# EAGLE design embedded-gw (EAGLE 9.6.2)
AUTHOR: Neal Jackson; REV: B; TITLE: Embedded GW

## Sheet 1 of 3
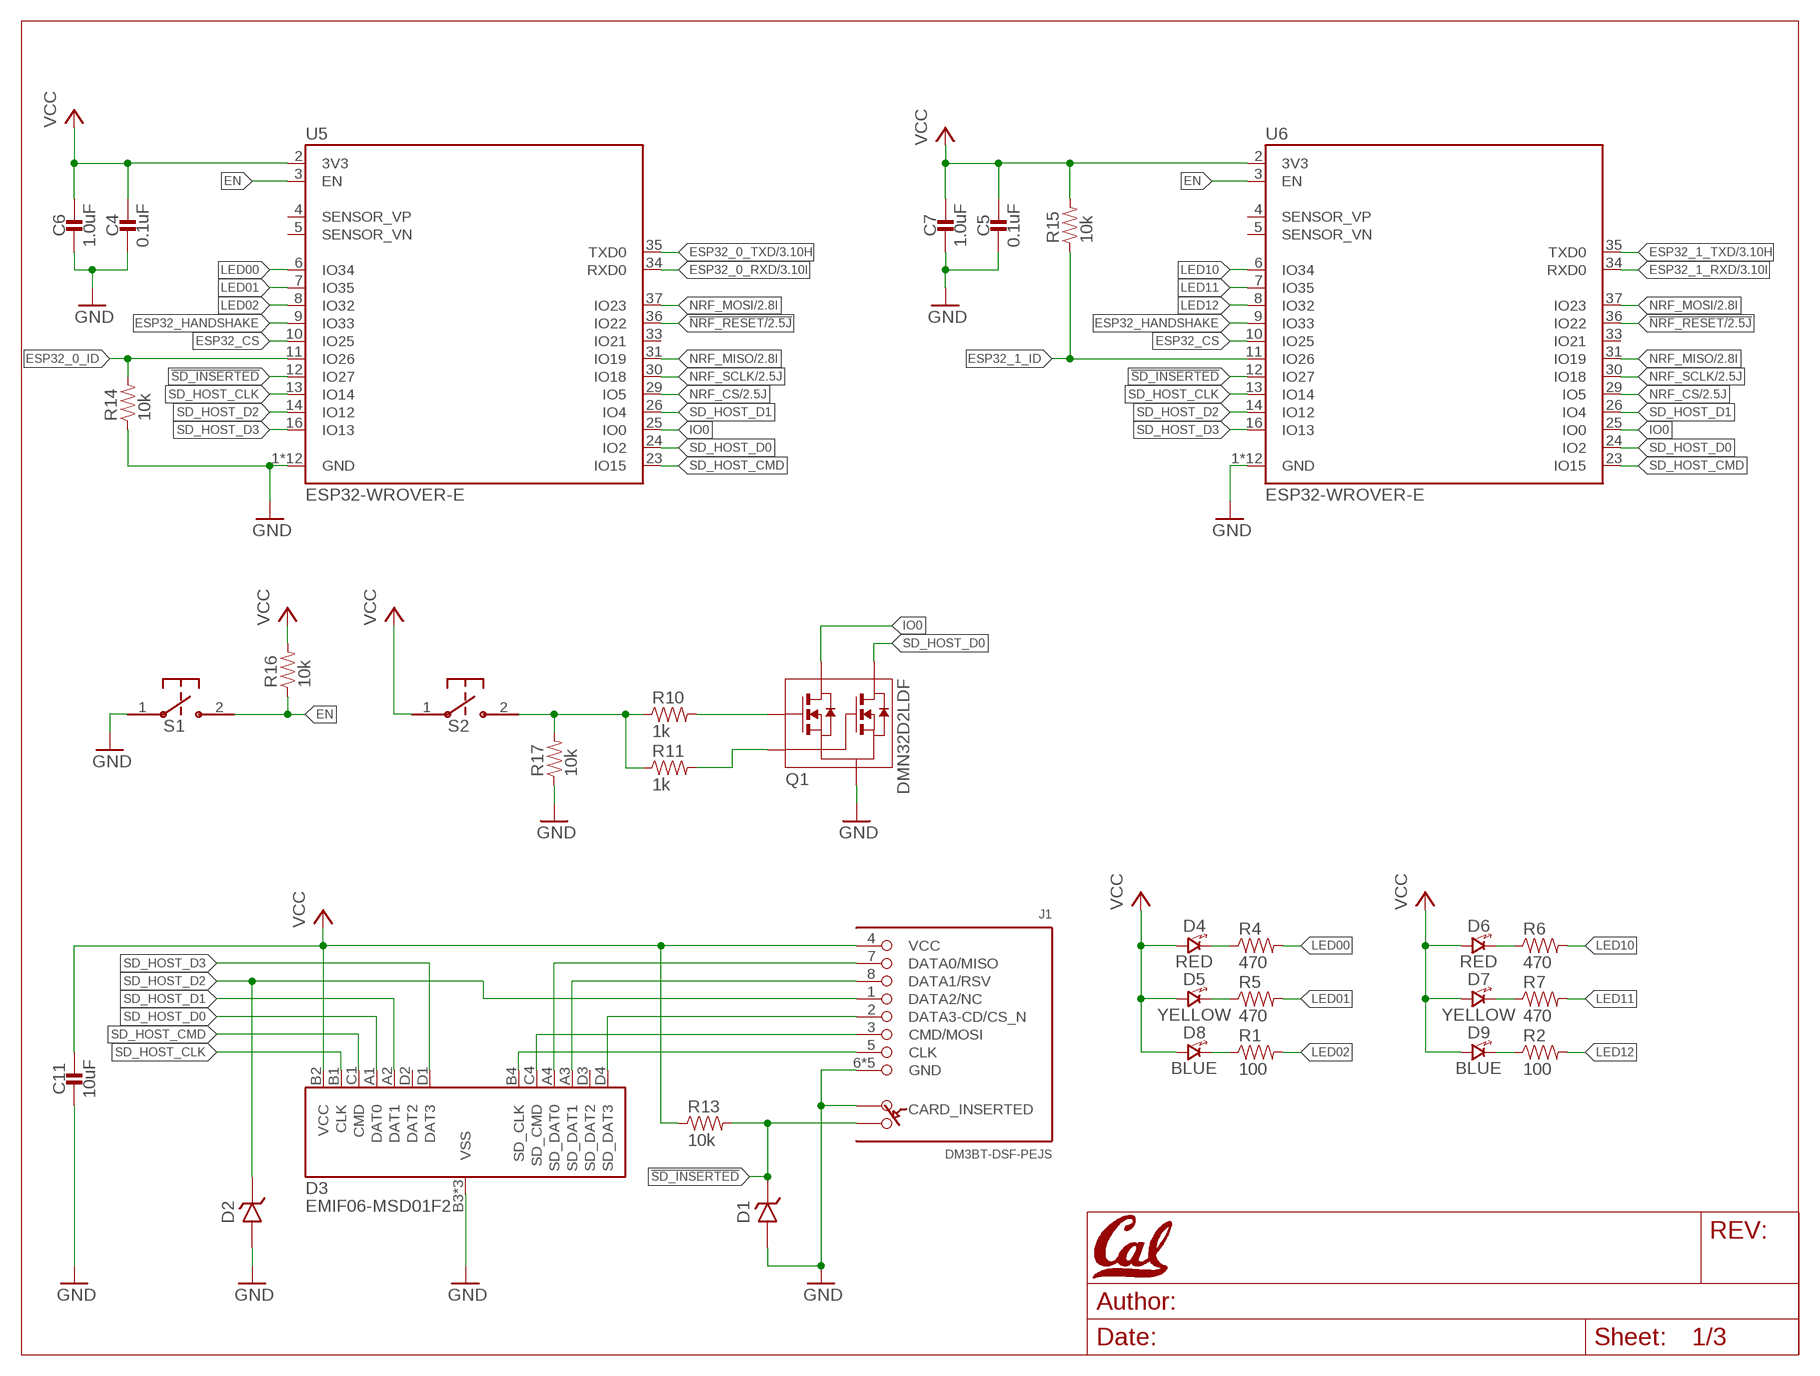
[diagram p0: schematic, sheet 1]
U$1 (LETTER_L_CAL): HEIGHT: 8.5in; WIDTH: 11in

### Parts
C4  0.1uF  CAPACITOR0402_CAP  [0402_CAP]
C5  0.1uF  CAPACITOR0402_CAP  [0402_CAP]
C6  1.0uF  CAPACITOR0402_CAP  [0402_CAP]
C7  1.0uF  CAPACITOR0402_CAP  [0402_CAP]
C11  10uF  CAPACITOR0805_CAP  [0805_CAP]
D1  DIODE_ZENER0201  [0201_DIODE]
D2  DIODE_ZENER0201  [0201_DIODE]
D3  EMIF06-MSD01F2  [BGA16C50P4X4_192X192X65N]
D4  RED  LED0603  [LED-0603]
D5  YELLOW  LED0603  [LED-0603]
D6  RED  LED0603  [LED-0603]
D7  YELLOW  LED0603  [LED-0603]
D8  BLUE  LED0603  [LED-0603]
D9  BLUE  LED0603  [LED-0603]
J1  DM3BT-DSF-PEJS  [HRS_DM3BT-DSF-PEJS]
Q1  DMN32D2LDF  [SOT353]
R1  100  RESISTOR0402_RES  [0402_RES]
R2  100  RESISTOR0402_RES  [0402_RES]
R4  470  RESISTOR0402_RES  [0402_RES]
R5  470  RESISTOR0402_RES  [0402_RES]
R6  470  RESISTOR0402_RES  [0402_RES]
R7  470  RESISTOR0402_RES  [0402_RES]
R10  1k  RESISTOR0402_RES  [0402_RES]
R11  1k  RESISTOR0402_RES  [0402_RES]
R13  10k  RESISTOR0402_RES  [0402_RES]
R14  10k  RESISTOR0402_RES  [0402_RES]
R15  10k  RESISTOR0402_RES  [0402_RES]
R16  10k  RESISTOR0402_RES  [0402_RES]
R17  10k  RESISTOR0402_RES  [0402_RES]
S1  B3U-1000P  [B3U-1000P]
S2  B3U-1000P  [B3U-1000P]
U5  ESP32-WROVER-E  [ESP32-WROVER-E]
U6  ESP32-WROVER-E  [ESP32-WROVER-E]

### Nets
!NRF_RESET: U5.36(IO22) U6.36(IO22) ; also sheet 2
!SD_INSERTED: D1.P$1(CATHODE) J1.SW-B(B) R13.2 U5.12(IO27) U6.12(IO27)
EN: R16.1 S1.2 U5.3(EN) U6.3(EN)
ESP32_0_ID: R14.2 U5.11(IO26)
ESP32_0_RXD: U5.34(RXD0) ; also sheet 3
ESP32_0_TXD: U5.35(TXD0) ; also sheet 3
ESP32_1_ID: R15.1 U6.11(IO26)
ESP32_1_RXD: U6.34(RXD0) ; also sheet 3
ESP32_1_TXD: U6.35(TXD0) ; also sheet 3
ESP32_CS: U5.10(IO25) U6.10(IO25)
ESP32_HANDSHAKE: U5.9(IO33) U6.9(IO33)
GND: C4.2 C5.2 C6.2 C7.2 C11.P$2 D1.P$2(ANODE) D2.P$2(ANODE) D3.B3(VSS) D3.C2(VSS) D3.C3(VSS) J1.6(GND) J1.S1(GND) J1.S2(GND) J1.S3(GND) J1.S4(GND) J1.SW-A(A) Q1.S R14.1 R17.1 S1.1 U5.1(GND) U5.15(GND) U5.38(GND) U5.GND1(GND) U5.GND2(GND) U5.GND3(GND) U5.GND4(GND) U5.GND5(GND) U5.GND6(GND) U5.GND7(GND) U5.GND8(GND) U5.GND9(GND) U6.1(GND) U6.15(GND) U6.38(GND) U6.GND1(GND) U6.GND2(GND) U6.GND3(GND) U6.GND4(GND) U6.GND5(GND) U6.GND6(GND) U6.GND7(GND) U6.GND8(GND) U6.GND9(GND) ; also sheet 2,3
IO0: Q1.D1 U5.25(IO0) U6.25(IO0)
LED00: R4.2 U5.6(IO34)
LED01: R5.2 U5.7(IO35)
LED02: R1.2 U5.8(IO32)
LED10: R6.2 U6.6(IO34)
LED11: R7.2 U6.7(IO35)
LED12: R2.2 U6.8(IO32)
N$1: Q1.G1 R10.2
N$4: Q1.G2 R11.2
N$5: R10.1 R11.1 R17.2 S2.2
N$6: D3.C4(SD_CMD) J1.3(CMD/MOSI)
N$8: D3.A4(SD_DAT0) J1.7(DATA0/MISO)
N$9: D3.A3(SD_DAT1) J1.8(DATA1/RSV)
N$11: D3.D4(SD_DAT3) J1.2(DATA3-CD/CS_N)
N$12: D4.C(CATHODE) R4.1
N$13: D3.B4(SD_CLK) J1.5(CLK)
N$14: D5.C(CATHODE) R5.1
N$15: D8.C(CATHODE) R1.1
N$19: D6.C(CATHODE) R6.1
N$20: D7.C(CATHODE) R7.1
N$21: D9.C(CATHODE) R2.1
NRF_CS: U5.29(IO5) U6.29(IO5) ; also sheet 2
NRF_MISO: U5.31(IO19) U6.31(IO19) ; also sheet 2
NRF_MOSI: U5.37(IO23) U6.37(IO23) ; also sheet 2
NRF_SCLK: U5.30(IO18) U6.30(IO18) ; also sheet 2
SD_HOST_CLK: D3.B1(CLK) U5.13(IO14) U6.13(IO14)
SD_HOST_CMD: D3.C1(CMD) U5.23(IO15) U6.23(IO15)
SD_HOST_D0: D3.A1(DAT0) Q1.D2 U5.24(IO2) U6.24(IO2)
SD_HOST_D1: D3.A2(DAT1) U5.26(IO4) U6.26(IO4)
SD_HOST_D2: D2.P$1(CATHODE) J1.1(DATA2/NC) U5.14(IO12) U6.14(IO12)
SD_HOST_D3: D3.D1(DAT3) U5.16(IO13) U6.16(IO13)
VCC: C4.1 C5.1 C6.1 C7.1 C11.P$1 D3.B2(VCC) D4.A(ANODE) D5.A(ANODE) D6.A(ANODE) D7.A(ANODE) D8.A(ANODE) D9.A(ANODE) J1.4(VCC) R13.1 R15.2 R16.2 S2.1 U5.2(3V3) U6.2(3V3) ; also sheet 2,3
Unconnected: D3.D2(DAT2) D3.D3(SD_DAT2) U5.4(SENSOR_VP) U5.5(SENSOR_VN) U5.33(IO21) U6.4(SENSOR_VP) U6.5(SENSOR_VN) U6.33(IO21)

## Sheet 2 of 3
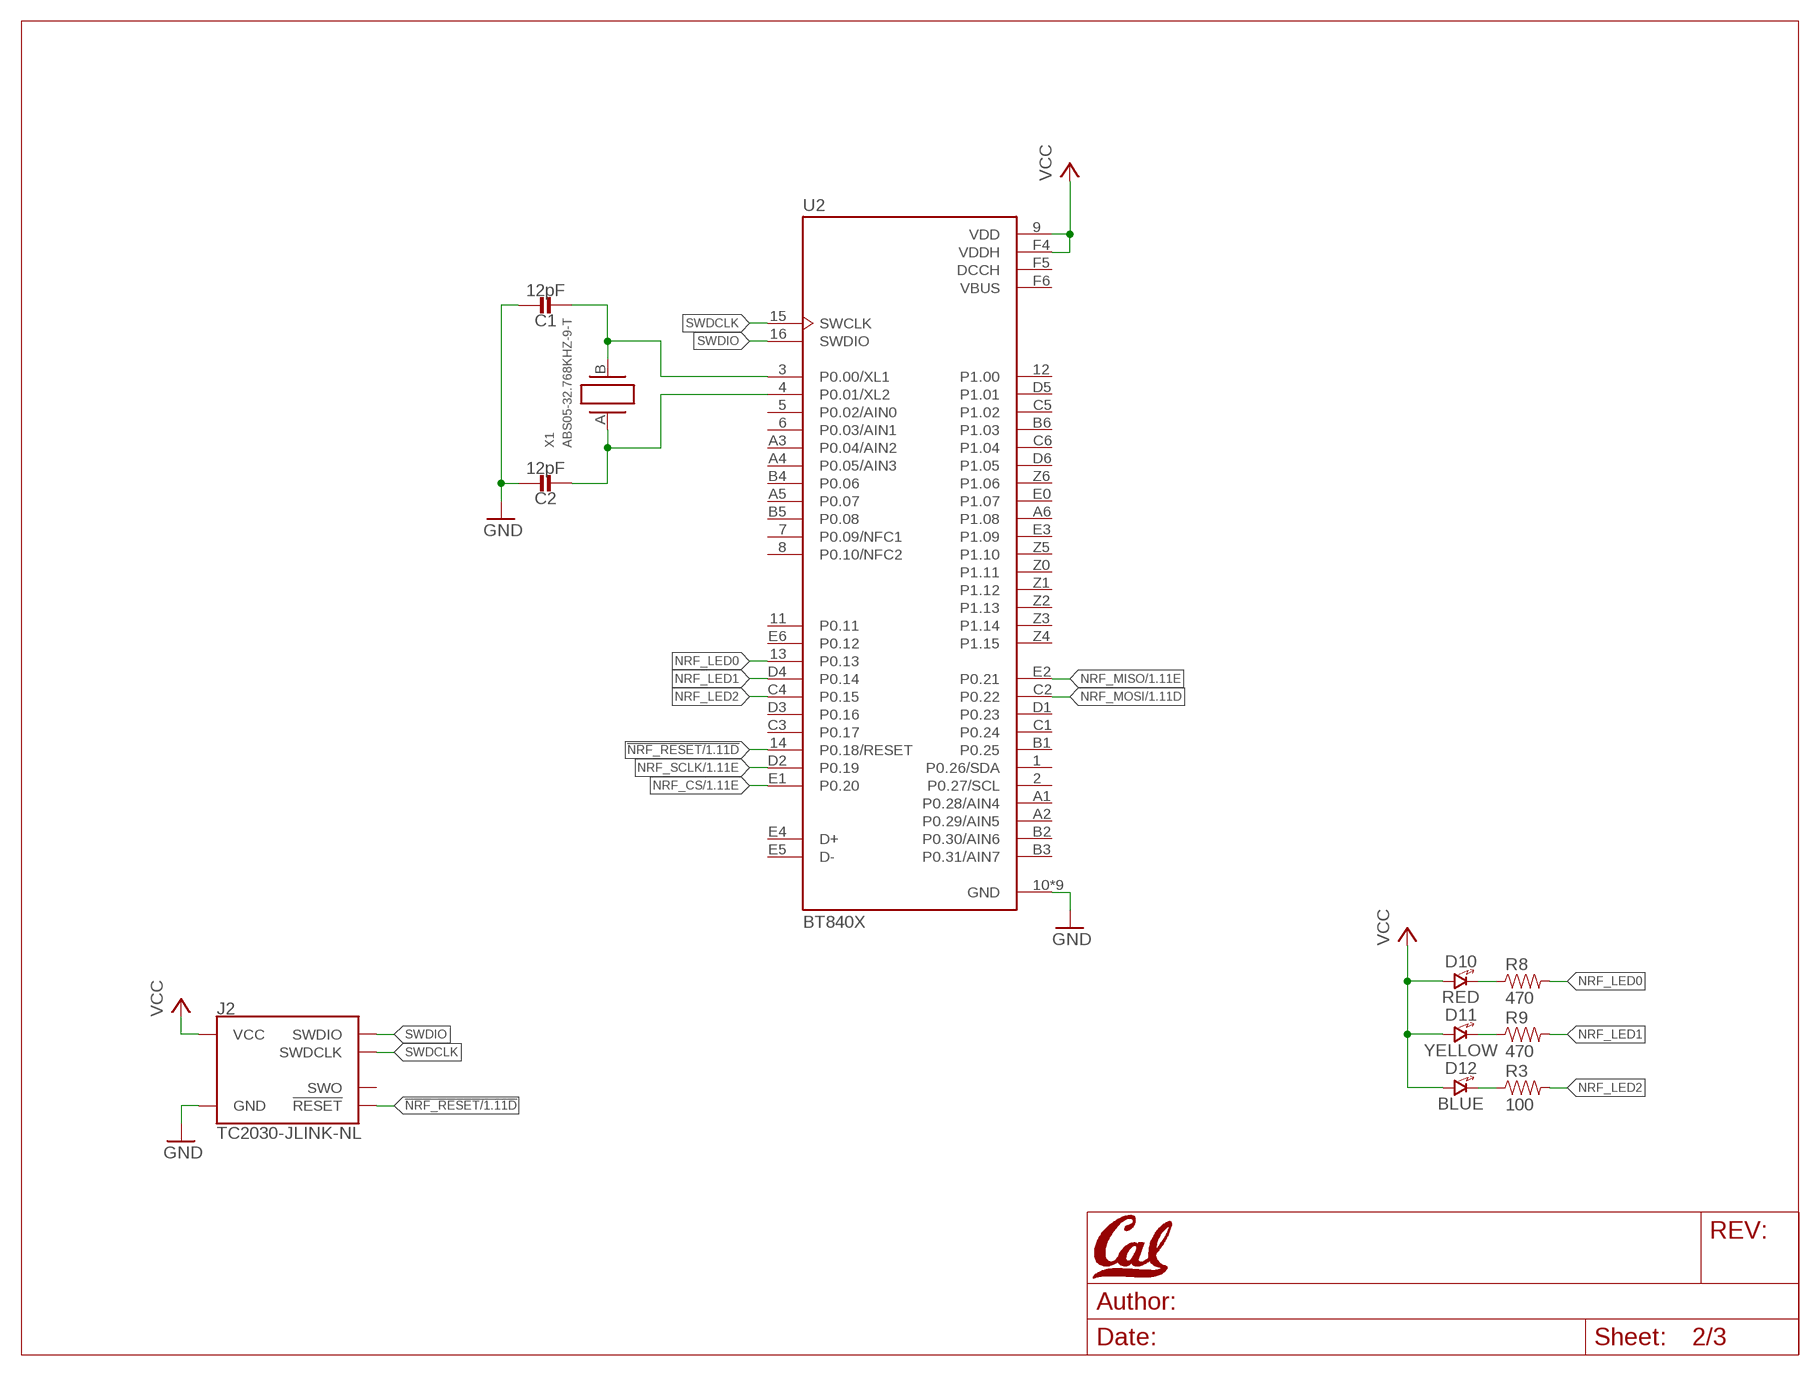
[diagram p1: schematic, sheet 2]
U$2 (LETTER_L_CAL): HEIGHT: 8.5in; WIDTH: 11in

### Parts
C1  12pF  CAPACITOR0402_CAP  [0402_CAP]
C2  12pF  CAPACITOR0402_CAP  [0402_CAP]
D10  RED  LED0603  [LED-0603]
D11  YELLOW  LED0603  [LED-0603]
D12  BLUE  LED0603  [LED-0603]
J2  TC2030-JLINK-NL  [TC2030-IDC-NL]
R3  100  RESISTOR0402_RES  [0402_RES]
R8  470  RESISTOR0402_RES  [0402_RES]
R9  470  RESISTOR0402_RES  [0402_RES]
U2  BT840X  [XCVR_BT840X]
X1  ABS05-32.768KHZ-9-T  [ABS05]

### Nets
!NRF_RESET: J2.3(!RESET) U2.14(P0.18/RESET) ; also sheet 1
GND: C1.1 C2.1 J2.5(GND) U2.10(GND) U2.A0(GND) U2.B0(GND) U2.C0(GND) U2.D0(GND) U2.F0(GND) U2.F1(GND) U2.F2(GND) U2.F3(GND) ; also sheet 1,3
N$2: C1.2 U2.3(P0.00/XL1) X1.B
N$3: C2.2 U2.4(P0.01/XL2) X1.A
N$22: D10.C(CATHODE) R8.1
N$23: D11.C(CATHODE) R9.1
N$24: D12.C(CATHODE) R3.1
NC: U2.F6(VBUS)
NRF_CS: U2.E1(P0.20) ; also sheet 1
NRF_LED0: R8.2 U2.13(P0.13)
NRF_LED1: R9.2 U2.D4(P0.14)
NRF_LED2: R3.2 U2.C4(P0.15)
NRF_MISO: U2.E2(P0.21) ; also sheet 1
NRF_MOSI: U2.C2(P0.22) ; also sheet 1
NRF_SCLK: U2.D2(P0.19) ; also sheet 1
SWDCLK: J2.4(SWDCLK) U2.15(SWCLK)
SWDIO: J2.2(SWDIO) U2.16(SWDIO)
VCC: D10.A(ANODE) D11.A(ANODE) D12.A(ANODE) J2.1(VCC) U2.9(VDD) U2.F4(VDDH) ; also sheet 1,3
Unconnected: J2.6(SWO) U2.1(P0.26/SDA) U2.2(P0.27/SCL) U2.5(P0.02/AIN0) U2.6(P0.03/AIN1) U2.7(P0.09/NFC1) U2.8(P0.10/NFC2) U2.11(P0.11) U2.12(P1.00) U2.A1(P0.28/AIN4) U2.A2(P0.29/AIN5) U2.A3(P0.04/AIN2) U2.A4(P0.05/AIN3) U2.A5(P0.07) U2.A6(P1.08) U2.B1(P0.25) U2.B2(P0.30/AIN6) U2.B3(P0.31/AIN7) U2.B4(P0.06) U2.B5(P0.08) U2.B6(P1.03) U2.C1(P0.24) U2.C3(P0.17) U2.C5(P1.02) U2.C6(P1.04) U2.D1(P0.23) U2.D3(P0.16) U2.D5(P1.01) U2.D6(P1.05) U2.E0(P1.07) U2.E3(P1.09) U2.E4(D+) U2.E5(D-) U2.E6(P0.12) U2.Z0(P1.11) U2.Z1(P1.12) U2.Z2(P1.13) U2.Z3(P1.14) U2.Z4(P1.15) U2.Z5(P1.10) U2.Z6(P1.06)

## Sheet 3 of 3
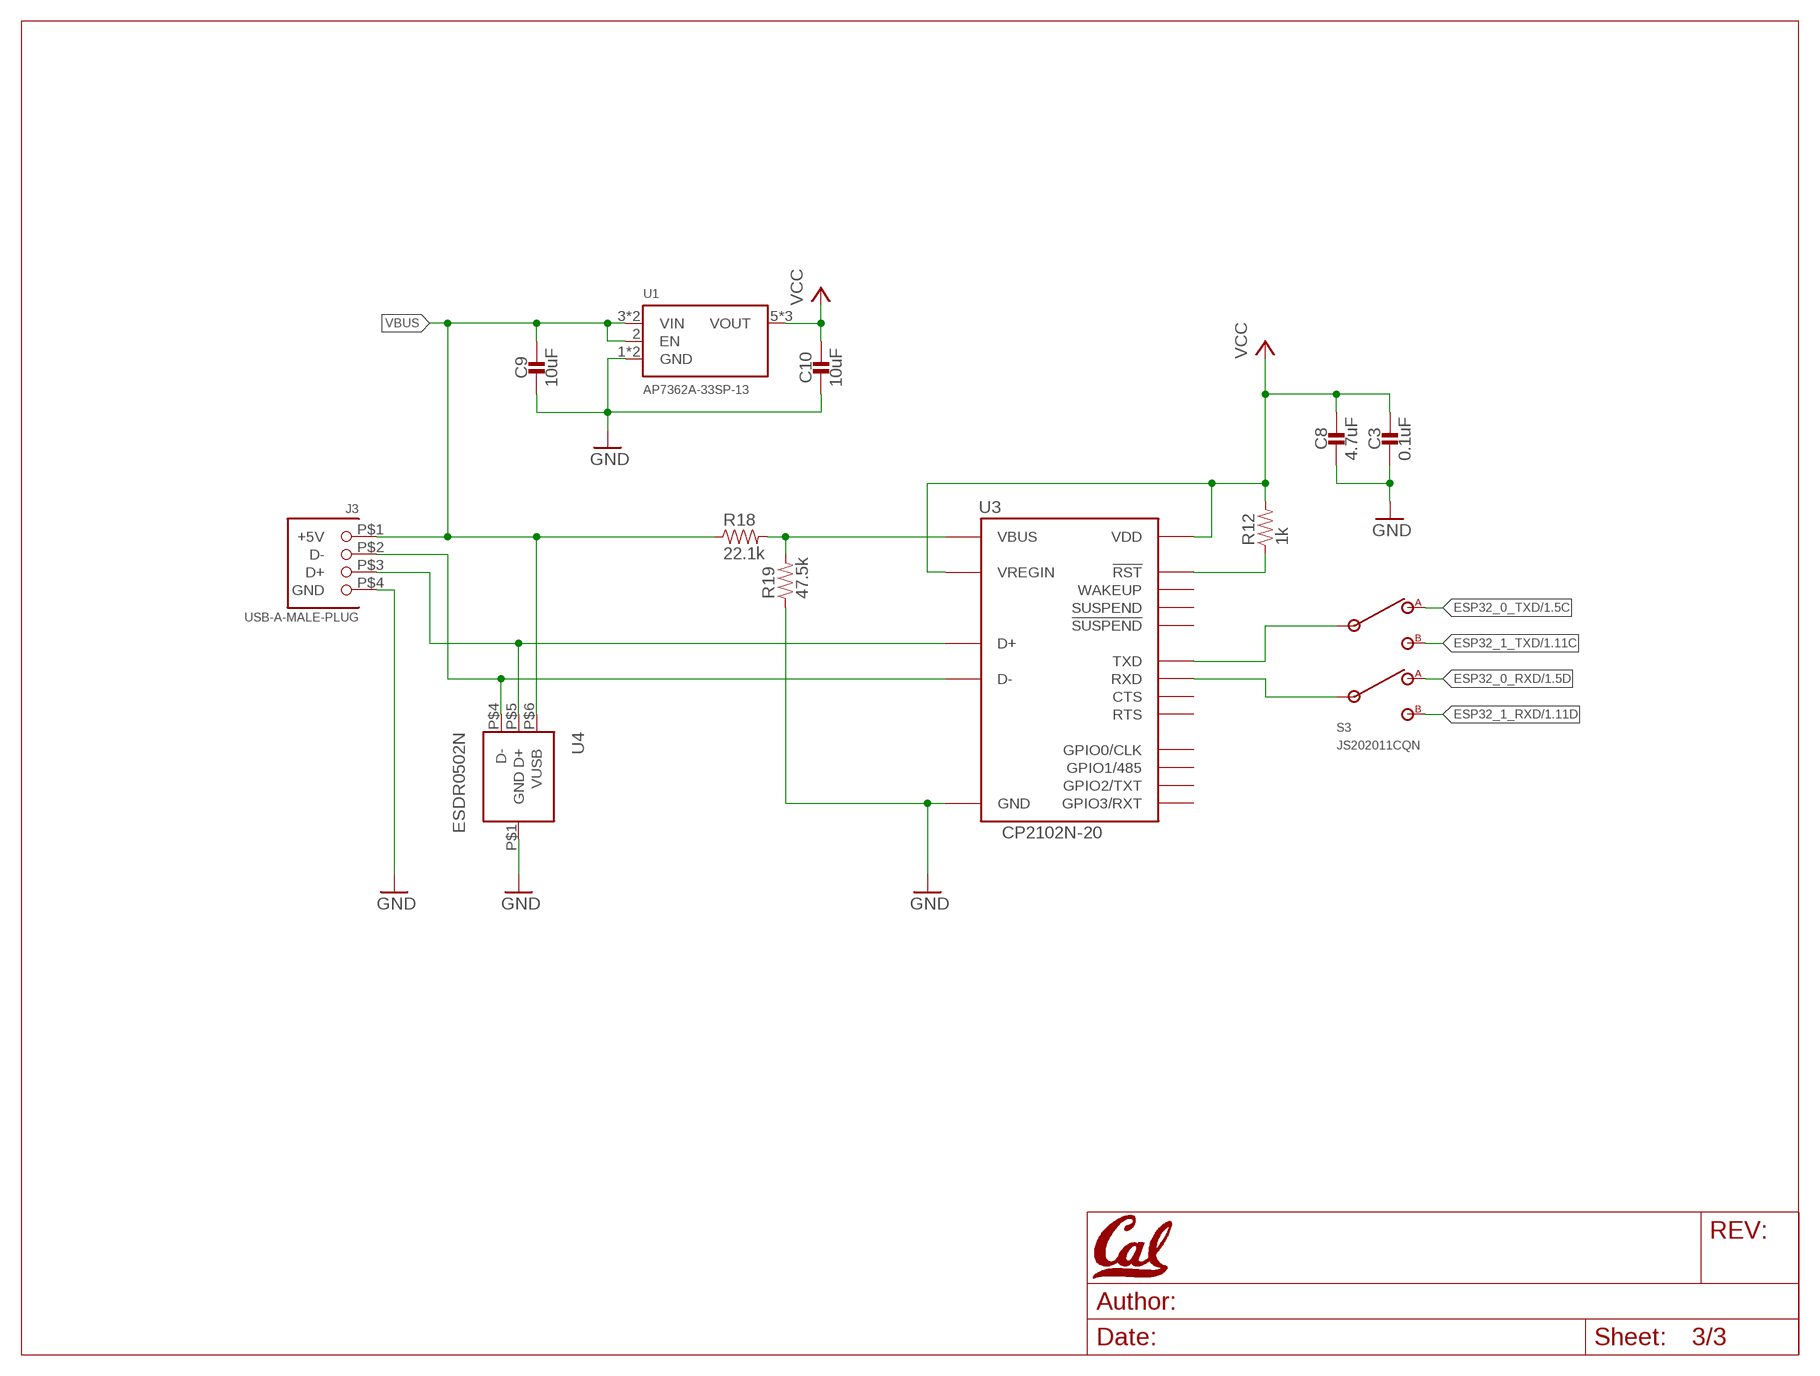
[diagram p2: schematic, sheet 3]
U$3 (LETTER_L_CAL): HEIGHT: 8.5in; WIDTH: 11in

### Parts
C3  0.1uF  CAPACITOR0402_CAP  [0402_CAP]
C8  4.7uF  CAPACITOR0603_CAP  [0603_CAP]
C9  10uF  CAPACITOR0805_CAP  [0805_CAP]
C10  10uF  CAPACITOR0805_CAP  [0805_CAP]
J3  USB-A-MALE-PLUG  [USB_A_MALE_PLUG_CUI_UP2-AH]
R12  1k  RESISTOR0402_RES  [0402_RES]
R18  22.1k  RESISTOR0402_RES  [0402_RES]
R19  47.5k  RESISTOR0402_RES  [0402_RES]
S3  JS202011CQN  [JS202011CQN]
U1  AP7362A-33SP-13  [SO-8EP]
U3  CP2102N-20  [QFN-20-3MM]
U4  ESDR0502N  [UDFN-6]

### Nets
D+: J3.P$3(D+) U3.4(D+) U4.P$5(D+)
D-: J3.P$2(D-) U3.5(D-) U4.P$4(D-)
ESP32_0_RXD: S3.1(A2) ; also sheet 1
ESP32_0_TXD: S3.4(A1) ; also sheet 1
ESP32_1_RXD: S3.3(B2) ; also sheet 1
ESP32_1_TXD: S3.6(B1) ; also sheet 1
GND: C3.2 C8.2 C9.P$2 C10.P$2 J3.P$4(GND) R19.1 U1.1(GND) U1.PAD(GND) U3.3(GND) U3.12(GND) U3.P$1(GND) U4.P$1(GND) ; also sheet 1,2
N$7: R12.1 U3.9(!RST)
N$10: R18.2 R19.2 U3.8(VBUS)
RXD: S3.2(I2) U3.17(RXD)
TXD: S3.5(I1) U3.18(TXD)
VBUS: C9.P$1 J3.P$1(+5V) R18.1 U1.2(EN) U1.3(VIN) U1.4(VIN) U4.P$6(VUSB)
VCC: C3.1 C8.1 C10.P$1 R12.2 U1.5(VOUT) U1.6(VOUT) U1.7(VOUT) U3.6(VDD) U3.7(VREGIN) ; also sheet 1,2
Unconnected: U3.1(GPIO1/485) U3.2(GPIO0/CLK) U3.11(!SUSPEND) U3.13(WAKEUP) U3.14(SUSPEND) U3.15(CTS) U3.16(RTS) U3.19(GPIO3/RXT) U3.20(GPIO2/TXT)

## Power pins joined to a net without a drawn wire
DCCH: U2.F5(DCCH)

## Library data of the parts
C1 C2 = passives:CAPACITOR: SMD Capacitor; DIGIKEY: 490-GCM1555C1H120GA16DCT-ND; MPN: GCM1555C1H120GA16D
C3-C5 = passives:CAPACITOR: SMD Capacitor; DIGIKEY: 1276-1511-1-ND; MPN: CL05B104KQ5NNNC
C6 C7 = passives:CAPACITOR: SMD Capacitor; DIGIKEY: 1276-1010-1-ND; MPN: CL05A105KQ5NNNC
C8 = passives:CAPACITOR: SMD Capacitor; DIGIKEY: 1276-1045-1-ND; MPN: CL10A475KQ8NNNC
C9-C11 = passives:CAPACITOR: SMD Capacitor; DIGIKEY: 1276-2404-1-ND; MPN: CL21A106KQCLNNC
D1 D2 = passives:DIODE_ZENER; DIGIKEY: ESD7381MUT5GOSCT-ND; MPN: ESD7381MUT5G
D3 = passives:EMIF06-MSD01F2: Mini and micro SD Card - EMI filtering and 25 kV ESD protection; DIGIKEY: 497-5903-1-ND; MANUFACTURER: STMicroelectronics; MPN: EMIF06-MSD01F2
D4 D6 D10 = leds:LED: LED; DIGIKEY: 160-1830-1-ND; MPN: LTST-C193KRKT-5A
D5 D7 D11 = leds:LED: LED; DIGIKEY: 160-1831-1-ND; MPN: LTST-C193KSKT-5A
D8 D9 D12 = leds:LED: LED; DIGIKEY: 160-1827-1-ND; MPN: LTST-C193TBKT-5A
J1 = connector:DM3BT-DSF-PEJS: 10 (8 + 2) Position Card Connector Secure Digital - microSD™ Surface Mount, Right Angle Gold Check prices; DIGIKEY: HR1942TR-ND; MANUFACTURER: Hirose Connector; MPN: DM3BT-DSF-PEJS
J2 = connector:TC2030-JLINK
J3 = connector:USB-A-MALE-PLUG: USB A Male plug connector; DIGIKEY: 102-3996-ND; MANUFACTURER: CUI; MPN: UP2-AH-1-TH
Q1 = fets:DMN32D2LDF: Common source dual n-channel mosfet; DIGIKEY: DMN32D2LDF-7DICT-ND; MANUFACTURER: Diodes Incorporated; MPN: DMN32D2LDF-7
R1-R3 = passives:RESISTOR: Resistor; DIGIKEY: 311-100JRCT-ND; MPN: RC0402JR-07100RL
R4-R9 = passives:RESISTOR: Resistor; DIGIKEY: 311-470LRCT-ND; MPN: RC0402FR-07470RL
R10-R12 = passives:RESISTOR: Resistor; DIGIKEY: RMCF0402JT1K00CT-ND; MPN: RMCF0402JT1K00
R13-R17 = passives:RESISTOR: Resistor; DIGIKEY: RMCF0402JT10K0CT-ND; MPN: RMCF0402JT10K0
R18 = passives:RESISTOR: Resistor; DIGIKEY: 311-22.1KLRCT-ND; MPN: RC0402FR-0722K1L
R19 = passives:RESISTOR: Resistor; DIGIKEY: 13-RT0402FRE0722K1LCT-ND; MPN: RT0402FRE0722K1L
S1 S2 = switches:B3U: Switch; DIGIKEY: SW1020CT-ND; MANUFACTURER: Omron; MPN: B3U-1000P
S3 = switches:JS202011CQN: DPDT through hole; DIGIKEY: 401-2001-ND; MANUFACTURER: C&K; MPN: JS202011CQN
U1 = chips:AP7362: The AP7362 is a 1.5A adjustable/fixed output voltage linear regulator with ultra-low dropout; DIGIKEY: AP7362A-33SP-13DICT-ND; MANUFACTURER: Diodes Incorporated; MPN: AP7362A-33SP-13
U2 = BT840X:BT840X: 802.15.4, Bluetooth Bluetooth v5.0, Thread, Zigbee® Transceiver Module 2.4GHz PCB Trace Surface Mou Check prices; DIGIKEY: 1914-BT840XCT-ND; MANUFACTURER: Fanstel Corp.; MPN: BT840X
U3 = chips:CP2102N-20: A cheap, simple USB to UART adapter; DIGIKEY: 336-3692-ND; MANUFACTURER: SiLabs; MPN: CP2102N-A01-GQFN20
U4 = chips:ESDR0502N; DIGIKEY: ESDR0502NMUTBGOSCT-ND; MPN: ESDR0502NMUTBG
U5 U6 = chips:ESP32-WROVER-E; DIGIKEY: 1965-ESP32-WROVER-E(8MB)CT-ND; MANUFACTURER: Espressif Systems; MPN: ESP32-WROVER-E (8MB)
X1 = crystals:ABS05-32.768KHZ: 32.768kHz Crystal; DIGIKEY: 535-11897-1-ND; MANUFACTURER: Abracon; MPN: ABS05-32.768KHZ-9-T

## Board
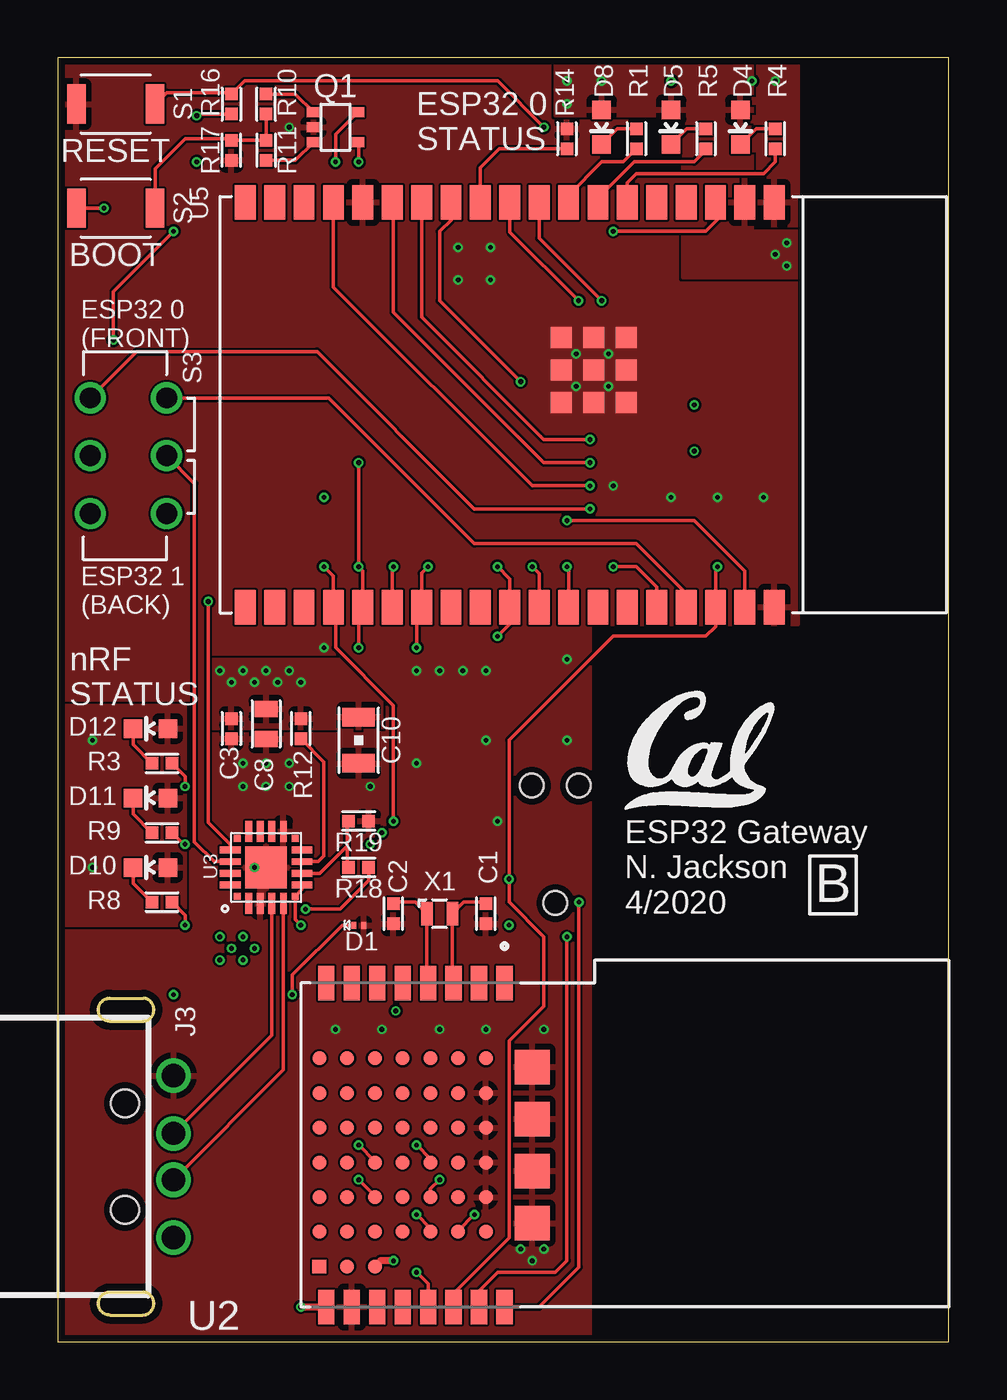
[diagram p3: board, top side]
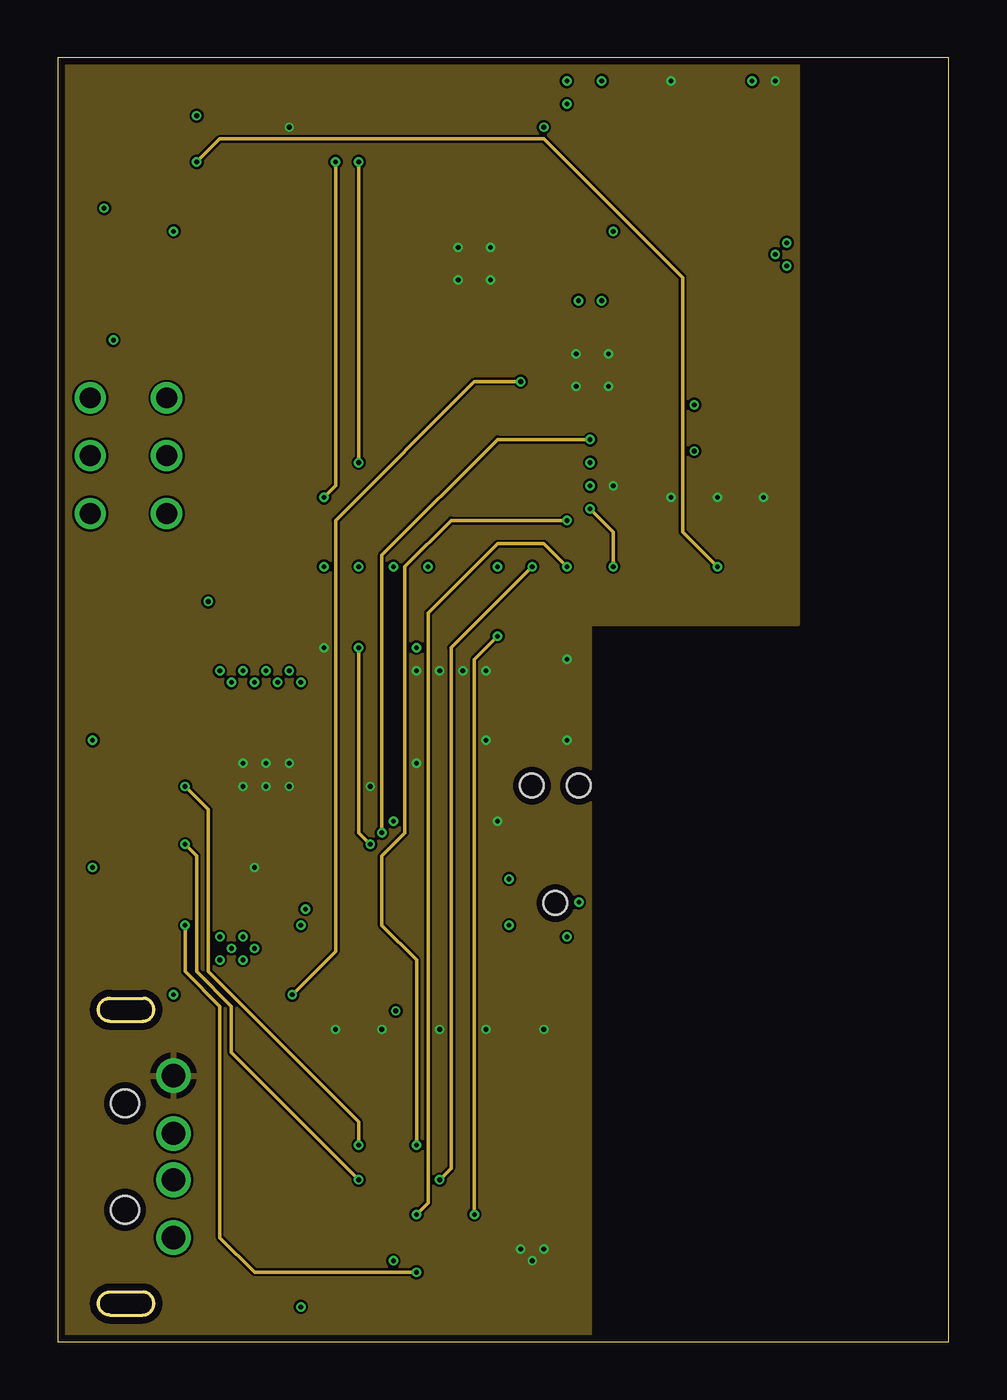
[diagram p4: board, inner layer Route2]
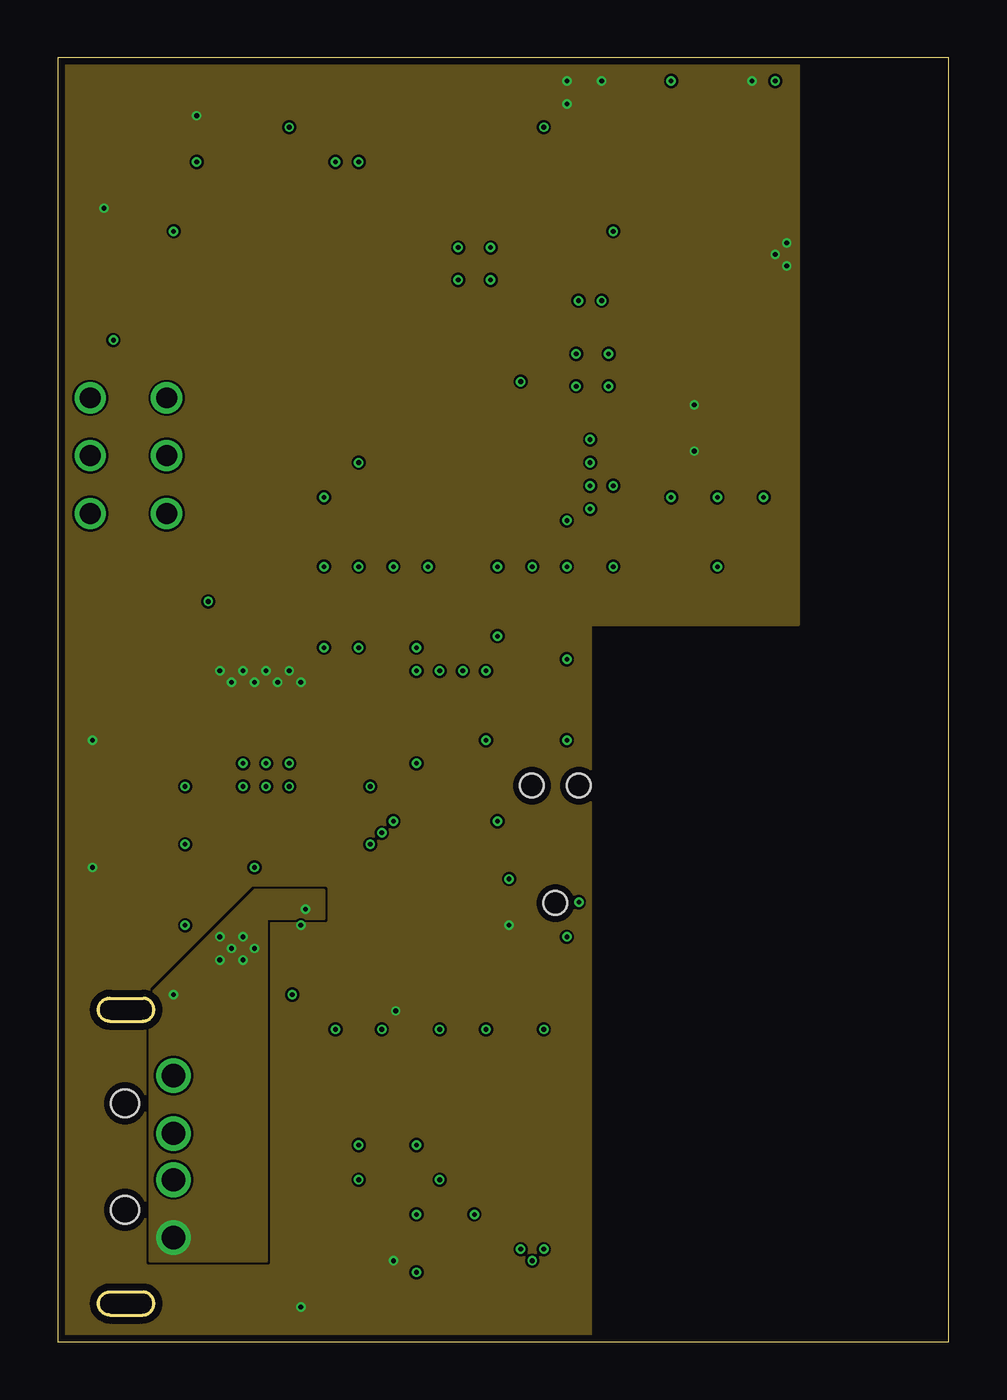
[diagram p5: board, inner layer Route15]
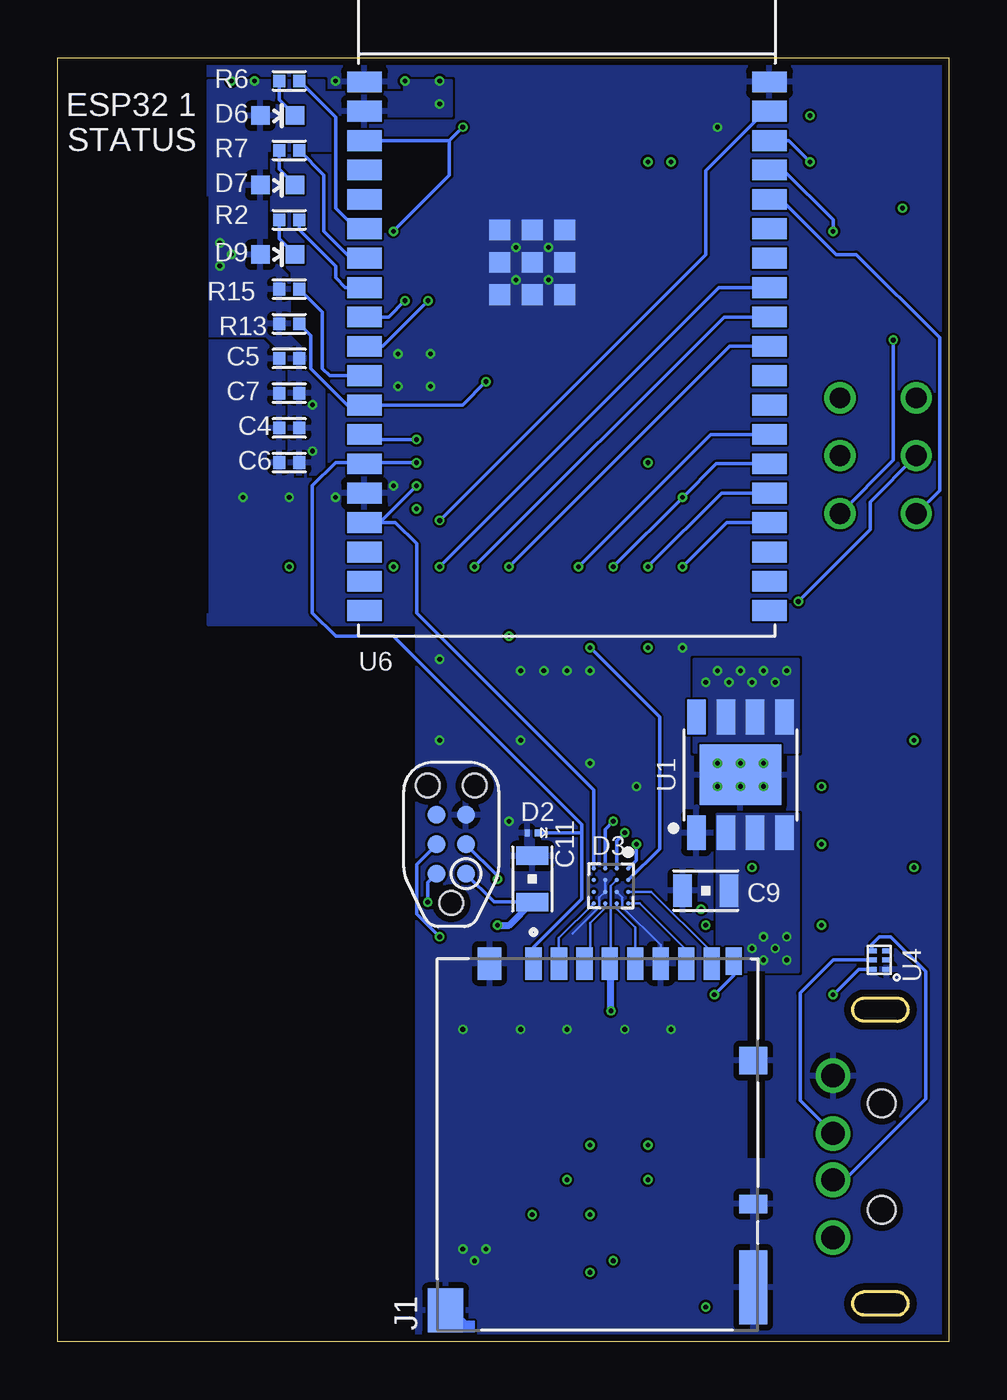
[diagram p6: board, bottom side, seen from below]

Size 38.5 x 55.5 mm. Coordinates in mm from the lower left corner, seen from the top.
Outline: 0,0 38.5,0 38.5,55.5 0,55.5 0,0
Copper layers (1+2*15+16): Top 0.0178mm / dielectric 59mil / Route2 0.0356mm / dielectric 0.1499mm / Route15 0.0356mm / dielectric 0.2007mm / Bottom 0.0178mm
Design rules "quickturn_co_kr_1oz_4lyr *": minimum track width 4mil, minimum drill 8mil, track to track 4mil, track to pad 4mil, pad to pad 4mil, via to via 4mil, smd to smd 4mil, copper to edge 12mil, drill to drill 12mil, minimum pad ring 8mil, minimum via ring 4mil, stop-mask expansion 3mil, vias tented up to drill 50mil, thermal gap 10mil

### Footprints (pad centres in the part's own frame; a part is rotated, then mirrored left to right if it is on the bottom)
0402_CAP = smd 0.536 x 0.546: 1 -0.433,0; 2 0.433,0
0603_CAP = smd 0.7 x 1: 1 -0.65,0; 2 0.65,0
0805_CAP = smd 0.8 x 1.4: P$1 1,0; P$2 -1,0
0201_DIODE = smd 0.3 x 0.21: P$1 0,0.22; P$2 0,-0.22
BGA16C50P4X4_192X192X65N = smd 0.2 x 0.2: A1 -0.75,0.75; A2 -0.25,0.75; A3 0.25,0.75; A4 0.75,0.75; B1 -0.75,0.25; B2 -0.25,0.25; B3 0.25,0.25; B4 0.75,0.25; C1 -0.75,-0.25; C2 -0.25,-0.25; C3 0.25,-0.25; C4 0.75,-0.25; D1 -0.75,-0.75; D2 -0.25,-0.75; D3 0.25,-0.75; D4 0.75,-0.75
LED-0603 = smd 0.8 x 0.8: A 0,-0.75; C 0,0.75
HRS_DM3BT-DSF-PEJS = smd 0.7 x 1.4: 1 -2.775,0.7; 2 -1.675,0.7; 3 -0.575,0.7; 4 0.525,0.7; 5 1.625,0.7; 6 2.725,0.7; 7 3.825,0.7; 8 4.925,0.7 | smd 1 x 1.4: S1 -4.675,0.7 | smd 1.2 x 1.2: S2 6.725,-3.5 | smd 1.2 x 3.2: S3 6.725,-13.3 | smd 1.5 x 1.9: S4 -6.575,-14.3 | smd 1.2 x 0.8: SW-A 6.725,-9.7 | smd 0.7 x 1.2: SW-B 5.875,0.8
TC2030-IDC-NL = smd 0.787 x 0.787: 1 -1.27,-0.635; 2 -1.27,0.635; 3 0,-0.635; 4 0,0.635; 5 1.27,-0.635; 6 1.27,0.635 | hole 1.016: -2.54,0; 2.54,1.016; 2.54,-1.016
USB_A_MALE_PLUG_CUI_UP2-AH = drill 1: P$1 3.5,5; P$2 1,5; P$3 -1,5; P$4 -3.5,5 | hole 1.2: -2.3,2.9; 2.3,2.9
SOT353 = smd 0.42 x 0.6: D1 0.65,-0.95; D2 -0.65,-0.95; G1 0.65,0.95; G2 -0.65,0.95; S 0,0.95
0402_RES = smd 0.536 x 0.546: 1 -0.433,0; 2 0.433,0
B3U-1000P = smd 0.8 x 1.7: 1 -1.7,0; 2 1.7,0
JS202011CQN = drill 0.9: 1 0,0; 2 2.5,0; 3 5,0; 4 0,3.3; 5 2.5,3.3; 6 5,3.3
SO-8EP = smd 1.505 x 0.802: 1 -2.5,1.905; 2 -2.5,0.635; 3 -2.5,-0.635; 4 -2.5,-1.905; 5 2.5,0.635; 6 2.5,-0.635; 7 2.5,-1.905; 8 2.5,1.905 | smd 2.613 x 3.502: PAD 0,0
XCVR_BT840X = smd 1.5 x 0.7: 1 -7,-5.2; 2 -7,-6.3; 3 -7,-7.4; 4 -7,-8.5; 5 -7,-9.6; 6 -7,-10.7; 7 -7,-11.8; 8 -7,-12.9; 9 7,-12.9; 10 7,-11.8; 11 7,-10.7; 12 7,-9.6; 13 7,-8.5; 14 7,-7.4; 15 7,-6.3; 16 7,-5.2 | smd 0.6 x 0.6: A0 -2.25,-6; A1 -2.25,-7.2; A2 -2.25,-8.4; A3 -2.25,-9.6; A4 -2.25,-10.8; A5 -2.25,-12; A6 -2.25,-13.2; B0 -0.75,-6; B1 -0.75,-7.2; B2 -0.75,-8.4; B3 -0.75,-9.6; B4 -0.75,-10.8; B5 -0.75,-12; B6 -0.75,-13.2; C0 0.75,-6; C1 0.75,-7.2; C2 0.75,-8.4; C3 0.75,-9.6; C4 0.75,-10.8; C5 0.75,-12; C6 0.75,-13.2; D0 2.25,-6; D1 2.25,-7.2; D2 2.25,-8.4; D3 2.25,-9.6; D4 2.25,-10.8; D5 2.25,-12; D6 2.25,-13.2; E0 3.75,-6; E1 3.75,-7.2; E2 3.75,-8.4; E3 3.75,-9.6; E4 3.75,-10.8; E5 3.75,-12; E6 3.75,-13.2; F4 5.25,-10.8; F5 5.25,-12; F6 5.25,-13.2; Z0 -3.75,-6; Z1 -3.75,-7.2; Z2 -3.75,-8.4; Z3 -3.75,-9.6; Z4 -3.75,-10.8; Z5 -3.75,-12; Z6 -3.75,-13.2 | smd 1.5 x 1.5: F0 -3.375,-4; F1 -1.125,-4; F2 1.125,-4; F3 3.375,-4
QFN-20-3MM = smd 0.3 x 0.3: 1 -1.25,1.25; 6 -1.25,-1.25; 11 1.25,-1.25; 16 1.25,1.25 | smd 0.9 x 0.3: 2 -1.55,0.75; 3 -1.55,0.25; 4 -1.55,-0.25; 5 -1.55,-0.75; 12 1.55,-0.75; 13 1.55,-0.25; 14 1.55,0.25; 15 1.55,0.75 | smd 0.3 x 0.9: 7 -0.75,-1.55; 8 -0.25,-1.55; 9 0.25,-1.55; 10 0.75,-1.55; 17 0.75,1.55; 18 0.25,1.55; 19 -0.25,1.55; 20 -0.75,1.55 | smd 1.8 x 1.8: P$1 0,0
UDFN-6 = smd 0.42 x 0.22: P$1 -0.325,0.4; P$2 -0.325,0; P$3 -0.325,-0.4; P$4 0.325,-0.4; P$5 0.325,0; P$6 0.325,0.4
ESP32-WROVER-E = smd 1.5 x 0.9: 1 0.25,23.96; 2 0.25,22.69; 3 0.25,21.42; 4 0.25,20.15; 5 0.25,18.88; 6 0.25,17.61; 7 0.25,16.34; 8 0.25,15.07; 9 0.25,13.8; 10 0.25,12.53; 11 0.25,11.26; 12 0.25,9.99; 13 0.25,8.72; 14 0.25,7.45; 15 0.25,6.18; 16 0.25,4.91; 17 0.25,3.64; 18 0.25,2.37; 19 0.25,1.1; 20 17.75,1.1; 21 17.75,2.37; 22 17.75,3.64; 23 17.75,4.91; 24 17.75,6.18; 25 17.75,7.45; 26 17.75,8.72; 27 17.75,9.99; 28 17.75,11.26; 29 17.75,12.53; 30 17.75,13.8; 31 17.75,15.07; 32 17.75,16.34; 33 17.75,17.61; 34 17.75,18.88; 35 17.75,20.15; 36 17.75,21.42; 37 17.75,22.69; 38 17.75,23.96 | smd 0.9 x 0.9: GND1 6.1,17.56; GND2 7.5,17.56; GND3 8.9,17.56; GND4 6.1,16.16; GND5 7.5,16.16; GND6 8.9,16.16; GND7 6.1,14.76; GND8 7.5,14.76; GND9 8.9,14.76
ABS05 = smd 0.5 x 1: A -0.55,0; B 0.55,0

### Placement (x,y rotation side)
C1  18.5,18.5 90 top
C2  14.5,18.5 90 top
C3  7.5,26.5 270 top
C4  28.5,39.5 180 bottom
C5  28.5,42.5 180 bottom
C6  28.5,38 180 bottom
C7  28.5,41 180 bottom
C8  9,26.7 270 top
C9  10.5,19.5 0 bottom
C10  13,26 90 top
C11  18,20 270 bottom
D1  13,18 90 top
D2  18,22 270 bottom
D3  14.6,19.7 270 bottom
D4  29.5,52.5 180 top
D5  26.5,52.5 180 top
D6  29,53 270 bottom
D7  29,50 270 bottom
D8  23.5,52.5 180 top
D9  29,47 270 bottom
D10  4,20.5 90 top
D11  4,23.5 90 top
D12  4,26.5 90 top
J1  15.17,15.65 0 bottom
J2  21.5,21.5 90 bottom
J3  0,8 270 top
Q1  12,52.5 90 top
R1  25,52 270 top
R2  28.5,48.5 0 bottom
R3  4.5,25 0 top
R4  31,52 270 top
R5  28,52 270 top
R6  28.5,54.5 0 bottom
R7  28.5,51.5 0 bottom
R8  4.5,19 0 top
R9  4.5,22 0 top
R10  9,53.5 90 top
R11  9,51.5 270 top
R12  10.5,26.5 90 top
R13  28.5,44 0 bottom
R14  22,52 270 top
R15  28.5,45.5 180 bottom
R16  7.5,53.5 270 top
R17  7.5,51.5 90 top
R18  13,20.5 180 top
R19  13,22.5 180 top
S1  2.5,53.5 0 top
S2  2.5,49 0 top
S3  1.4,40.8 270 top
U1  9,24.5 90 bottom
U2  24.5,8.5 270 top
U3  9,20.5 90 top
U4  3,16.5 180 bottom
U5  7,49.5 270 top
U6  25.5,30.5 0 bottom
U$4  [UCB_CAL_200MIL]  24.5,23 0 top
X1  16.5,18.5 0 top

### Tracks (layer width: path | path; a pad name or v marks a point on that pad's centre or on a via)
!NRF_RESET  (via drill 0.2)
  Top 0.152: v28.5,33.5 28.42,33.42 U5.36 28.42,30.92 28,30.5 24,30.5 19.5,26 v19.5,20 19.5,19 21,17.5 21,14.5 19.5,13 19.5,4.5 17.1,2.1 U2.14
  Route2 0.152: v6,51 7,52 21,52 27,46 27,35 v28.5,33.5
  Bottom 0.152: v19.5,20 19.5,20.14 J2.3 | U6.36 6.92,51.92 v6,51
!SD_INSERTED  (via drill 0.2)
  Top 0.152: U5.12 16.99,48.49 16.5,48 16.5,45 v20,41.5 | v10.13,15 10.13,15.85 12.28,18 D1.P$1
  Route2 0.152: v20,41.5 18,41.5 12,35.5 12,16.87 v10.13,15
  Bottom 0.152: J1.SW-B 9.29,15.84 v10.13,15 | v20,41.5 21.01,40.49 U6.12 25.99,40.49 27.57,42.07 27.57,43.5 R13.2
D+
  Top 0.152: U3.4 9.25,13.25 J3.P$3
  Bottom 0.152: U4.P$5 5,16.5 6.43,15.07 6.43,10.43 J3.P$3
D-
  Top 0.152: U3.5 9.75,11.75 J3.P$2
  Bottom 0.152: U4.P$4 3.33,17.18 3,17.5 2.5,17.5 1,16 1,10.5 4.5,7 J3.P$2
EN  (via drill 0.2)
  Top 0.102: 28.5,48.5 28.5,49.17 U5.3
  Top 0.152: S1.2 4.7,54 7.43,54 R16.1 8.07,54.5 19,54.5 v21,52.5 | v24,48 28,48 28.5,48.5
  Bottom 0.152: v21,52.5 21.58,51.92 | 21.58,51.92 U6.3 | v24,48 21.58,50.42 21.58,51.92
ESP32_0_ID
  Top 0.152: U5.11 18.26,50.76 19.07,51.57 R14.2
ESP32_0_RXD  (via drill 0.2)
  Top 0.152: v24,33.5 25,33.5 25.88,32.62 U5.34 | v23,36 18,36 11.2,42.8 3.4,42.8 S3.1
  Route2 0.152: v23,36 24,35 v24,33.5
ESP32_0_TXD
  Top 0.152: U5.35 27.15,32.35 25,34.5 18,34.5 11.7,40.8 S3.4
ESP32_1_ID
  Bottom 0.152: U6.11 26.76,41.76 27.07,42.07 27.07,44.5 R15.1
ESP32_1_RXD
  Bottom 0.152: U6.34 7.25,49.38 4.87,47 4,47 0.4,43.4 0.4,36.8 S3.3
ESP32_1_TXD  (via drill 0.2)
  Top 0.152: v5,48 2.4,45.4 v2.4,43.3
  Bottom 0.152: U6.35 7.15,50.65 5,48.5 v5,48 | v2.4,43.3 2.4,38.1 S3.6
ESP32_CS  (via drill 0.2)
  Top 0.152: U5.10 19.53,47.97 v22.5,45
  Bottom 0.152: U6.10 24.47,43.03 v22.5,45
ESP32_HANDSHAKE  (via drill 0.2)
  Top 0.152: U5.9 20.8,47.7 v23.5,45
  Bottom 0.152: v23.5,45 24.2,44.3 U6.9
GND  (via drill 0.2)
  Bottom 0.102: J1.6 12.45,17.14 14.1,18.8 14.1,19.2 D3.B3 | D3.C2 D3.C3 15.1,19.2 15.1,18.8 16.25,17.65
  other vias: 8,25 9,25 10,25 8,24 9,24 10,24 8.5,20.5 20,4 21,4 20.5,3.5 21,13.5 18.5,13.5 11.5,30 17.3,47.3 18.7,47.3 17.3,45.9 18.7,45.9 22.4,42.7 23.8,42.7 22.4,41.3 23.8,41.3 13.5,24 31,54.5 26.5,54.5 14,13.5 19,22.5 22,26 15.5,25 26.5,36.5 24,37 28.5,36.5 30.5,36.5 22,29.5 18.5,26 18.5,29 17.5,29 16.5,29 15.5,29 12,13.5 10,52.5 16.5,13.5
  pour Top (rank 2): 0,55.5 32,55.5 32,31 23,31 23,0 0,0
  pour Bottom (rank 2): 0,55.5 32,55.5 32,31 23,31 23,0 0,0
  pour Route2: 0,55.5 32,55.5 32,31 23,31 23,0 0,0
  pour Bottom (no thermals): 15.5,49 15.5,44 20.5,44 20.5,49
  pour Top (no thermals): 20.5,44.5 25.5,44.5 25.5,39.5 20.5,39.5
IO0  (via drill 0.2)
  Top 0.152: U5.25 14.45,33.45 v14.5,33.5 | Q1.D1 12,52.2 v12,51
  Route2 0.152: v12,51 12,37 v11.5,36.5
  Bottom 0.152: U6.25 10.05,37.95 v11.5,36.5 v14.5,33.5
LED00
  Top 0.152: U5.6 24.61,50.11 25,50.5 30.5,50.5 31,51 R4.2
LED01
  Top 0.152: R5.2 28,51.5 27.5,51 24.91,51 23.34,49.43 U5.7
LED02
  Top 0.152: U5.8 22.07,49.57 23.5,51 24.43,51 R1.2
LED10
  Bottom 0.152: U6.6 25.61,48.11 26.5,49 26.5,52.93 R6.2
LED11
  Bottom 0.152: R7.2 27,50.43 27,48 25.84,46.84 U6.7
LED12
  Bottom 0.152: R2.2 28.07,48.07 26.5,46.5 26.5,46 26.07,45.57 U6.8
N$1
  Top 0.152: R10.2 10.27,53.93 Q1.G1
N$2
  Top 0.152: U2.3 17.05,15.55 X1.B 17.55,19 18.43,19 C1.2
N$3
  Top 0.152: C2.2 14.57,19 15.45,19 X1.A 15.95,15.55 U2.4
N$4
  Top 0.152: R11.2 10.27,51.07 Q1.G2
N$5
  Top 0.152: S2.2 4.2,50.7 5.5,52 7.43,52 R17.2 R11.1 R10.1
N$6
  Bottom 0.102: J1.3 15.5,16.59 15.5,18.1 14.85,18.75 D3.C4
N$7
  Top 0.152: U3.9 11.25,20.75 11.5,21 11.5,25.07 R12.1
N$8
  Bottom 0.102: D3.A4 13.35,18.95 11.35,16.95 J1.7
N$9
  Bottom 0.102: D3.A3 12.85,19.45 10.24,16.84 J1.8
N$10
  Top 0.152: R19.2 12.5,22.43 12.5,21.5 12.5,21.43 | U3.8 11.32,20.25 12.5,21.43 | R18.2 12.5,20.57 12.5,21.43
N$11
  Bottom 0.102: J1.2 16.84,17.45 D3.D4
N$12
  Top 0.152: D4.C 30.18,52.43 R4.1
N$13
  Bottom 0.102: J1.5 13.54,17.9 14.35,18.7 D3.B4
N$14
  Top 0.152: D5.C 27.18,52.43 R5.1
N$15
  Top 0.152: D8.C 24.18,52.43 R1.1
N$19
  Bottom 0.152: R6.1 28.93,53.68 D6.C
N$20
  Bottom 0.152: R7.1 28.93,50.68 D7.C
N$21
  Bottom 0.152: D9.C 28.93,47.68 R2.1
N$22
  Top 0.152: R8.1 3.25,19.82 D10.C
N$23
  Top 0.152: R9.1 3.25,22.82 D11.C
N$24
  Top 0.152: R3.1 3.25,25.82 D12.C
NRF_CS  (via drill 0.2)
  Top 0.152: U2.E1 17.3,4.8 v18,5.5 | v19,33.5 19.53,32.97 U5.29 19.53,31.03 v19,30.5
  Route2 0.152: v19,30.5 18,29.5 v18,5.5
  Bottom 0.152: U6.29 9.47,43.03 v19,33.5
NRF_LED0  (via drill 0.2)
  Top 0.152: R8.2 5.5,18.43 v5.5,18 | U2.13 16,2.5 v15.5,3
  Route2 0.152: v15.5,3 8.5,3 7,4.5 7,14.5 5.5,16 v5.5,18
NRF_LED1  (via drill 0.2)
  Top 0.152: v13,7 13.7,6.3 U2.D4 | R9.2 5.43,21.5 v5.5,21.5
  Route2 0.152: v13,7 7.5,12.5 7.5,14.5 6,16 6,21 v5.5,21.5
NRF_LED2  (via drill 0.2)
  Top 0.152: v13,8.5 13.7,7.8 U2.C4 | R3.2 5.5,24.43 v5.5,24
  Route2 0.152: v5.5,24 6.5,23 6.5,16 13,9.5 v13,8.5
NRF_MISO  (via drill 0.2)
  Top 0.152: v15.5,5.5 16.1,4.9 U2.E2 | v22,33.5 22.07,33.43 U5.31
  Route2 0.152: v15.5,5.5 16,6 16,31.5 19,34.5 21,34.5 v22,33.5
  Bottom 0.152: U6.31 9.93,45.57 v22,33.5
NRF_MOSI  (via drill 0.2)
  Top 0.152: v15.5,8.5 16.1,7.9 U2.C2 | v22,35.5 27.5,35.5 29.69,33.31 U5.37
  Route2 0.152: v15.5,8.5 15.5,16.5 14,18 14,21 15,22 15,33.5 17,35.5 v22,35.5
  Bottom 0.152: U6.37 7.93,53.19 10.5,50.62 10.5,47 v22,35.5
NRF_SCLK  (via drill 0.2)
  Top 0.152: v16.5,7 16.1,6.6 U2.D2 | v20.5,33.5 20.8,33.2 U5.30
  Route2 0.152: v16.5,7 17,7.5 17,30 v20.5,33.5
  Bottom 0.152: U6.30 9.7,44.3 v20.5,33.5
RXD  (via drill 0.2)
  Top 0.152: U3.17 7.45,21.5 6.5,22.45 v6.5,32
  Bottom 0.152: S3.2 3.4,36.3 3.4,35.1 v6.5,32
SD_HOST_CLK  (via drill 0.2)
  Top 0.152: v23,39 21,39 15.72,44.28 U5.13
  Route2 0.152: v14,22 14,34 19,39 v23,39
  Bottom 0.152: D3.B1 14.35,21.65 v14,22 | U6.13 25.03,39 v23,39
SD_HOST_CMD  (via drill 0.2)
  Top 0.152: v11.5,33.5 11.91,33.09 U5.23 12,31.66 12,30 14.5,27.5 v14.5,22.5
  Bottom 0.152: D3.C1 14.85,22.15 v14.5,22.5 | U6.23 9.59,35.41 v11.5,33.5
SD_HOST_D0  (via drill 0.2)
  Top 0.152: v13,30 13,31.57 U5.24 13.18,33.32 v13,33.5 v13,38 | Q1.D2 13,51.8 v13,51
  Route2 0.152: v13.5,21.5 13,22 v13,30 | v13,51 v13,38
  Bottom 0.152: v13.5,21.5 13.5,20.8 D3.A1 | U6.24 9.82,36.68 v13,33.5
SD_HOST_D1  (via drill 0.2)
  Top 0.152: v16,33.5 15.72,33.22 U5.26 15.5,31.53 v15.5,30
  Bottom 0.152: U6.26 10.28,39.22 v16,33.5 | D3.A2 12.5,21.3 12.5,27 v15.5,30
SD_HOST_D2  (via drill 0.2)
  Top 0.152: U5.14 14.5,49.2 14.5,44.5 21,38 v23,38
  Bottom 0.152: v23,38 25.2,38 U6.14 25.3,38 26.5,38 27.5,37 27.5,31.5 26.5,30.5 24,30.5 15.85,22.35 15.85,22 | 15.85,22 15.85,19.15 17.95,17.05 J1.1 | D2.P$1 15.85,22
SD_HOST_D3  (via drill 0.2)
  Top 0.152: U5.16 11.91,45.59 20.5,37 v23,37
  Bottom 0.152: v23,37 24.59,35.41 U6.16 23.91,35.41 23,34.5 23,31.5 15.35,23.85 D3.D1
SWDCLK  (via drill 0.2)
  Top 0.152: U2.15 18.2,2.2 19,3 21.5,3 22,3.5 v22,17.5
  Bottom 0.152: v22,17.5 23,18.5 23,20.64 J2.4
SWDIO  (via drill 0.2)
  Top 0.152: U2.16 20.8,1.5 22.52,3.22 v22.52,19
  Bottom 0.152: v22.52,19 22.52,19.85 J2.2
TXD
  Top 0.152: U3.18 6.75,20.75 5.9,21.6 5.9,37.1 S3.5
VBUS  (via drill 0.2)
  Top 0.152: R18.1 13.43,19.93 12.2,18.7 v10.7,18.7
  Bottom 0.152: U4.P$6 3.9,16.1 v5,15
  other vias: 7,17.5 7,16.5 7.5,17 8,17.5 8.5,17 8,16.5
  pour Bottom (no thermals): 6.5,22.8 6.5,16 10,16 10,22.8
  pour Route15 (no thermals): 9,3.5 4,3.5 4,15 8.5,19.5 11.5,19.5 11.5,18.3 9,18.3
VCC  (via drill 0.2)
  Top 0.152: R16.2 6.07,53.07 v6,53 | S2.1 v2,49 | U3.7 10.55,19.55 U3.6 10.25,18.25 v10.5,18
  Top 0.305: v10.5,1.5 U2.9 | v14.5,3.5 13.95,3.5 U2.F4
  Bottom 0.102: D3.B2 14.6,19.7 14.6,16.39 J1.4
  Bottom 0.152: C11.P$1 19.64,19 J2.1
  Bottom 0.305: v19.5,18 19,18 C11.P$1 | v14.6,14.3 14.6,16.3 J1.4
  other vias: 7.5,28.5 8.5,28.5 8,29 9,29 30,54.5 23.5,54.5 31,47 31.5,47.5 31.5,46.5 1.5,26 1.5,20.5 22,54.5 22,53.5 27.5,40.5 27.5,38.5 9.5,28.5 10,29 10.5,28.5 7,29
  pour Route15 (rank 2): 0,55.5 32,55.5 32,31 23,31 23,0 0,0
  pour Bottom (no thermals): 11,29.5 6.5,29.5 6.5,25.5 11,25.5
  pour Top: 30,55.5 21.5,55.5 21.5,53 27,53 27,46 32,46 32,48 30,48
  pour Bottom: 32,54.5 27,54.5 27,54 23.5,54 23.5,54.5 21.5,54.5 21.5,53 24.5,53 24.5,51.5 29.5,51.5 29.5,47 28.5,46 28.5,43.5 27,42 27,37.5 28.5,37.5 28.5,42.5 29.5,43.5 32,43.5
  pour Top: 0,27.5 5.5,27.5 5.5,18 0,18
  pour Top: 6.5,29.5 6.5,26.5 14,26.5 14,29.5

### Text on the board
tPlace: ESP32 0 / STATUS | ESP32 0 / (FRONT) | ESP32 1 / (BACK) | nRF / STATUS | ESP32 Gateway / N. Jackson / 4/2020
bPlace: ESP32 1 / STATUS
tNames: RESET | BOOT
